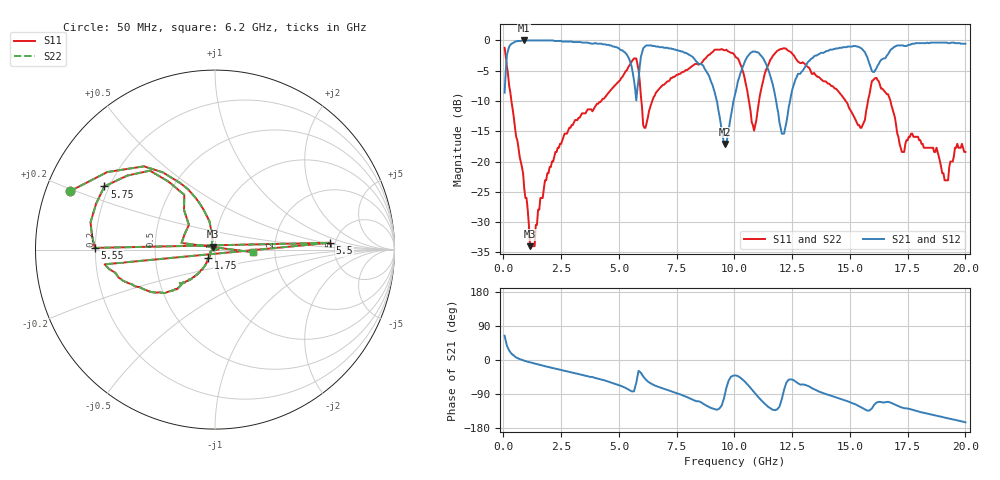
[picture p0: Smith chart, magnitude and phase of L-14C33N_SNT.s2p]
#	mhz	s	ma	r	50
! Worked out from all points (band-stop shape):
!   400 points, 50 MHz to 20 GHz, reference 50 ohm
!   highest |S21| = 0.00 dB at 900 MHz (marker M1); lowest = -17.1 dB at 9.6 GHz (marker M2)
!   |S21| within 3 dB of the highest: 138.4 MHz to 5.437 GHz (5.298 GHz wide, 190 % of centre); 16.44 GHz to end of sweep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
!   lowest |S11| = -34.0 dB at 1.15 GHz (marker M3), VSWR 1.04, Z = 48.7 + j1.52 ohm
!   |S11| at or under -10 dB: 344.4 MHz to 4.231 GHz (3.887 GHz wide, 170 % of centre); 14.82 GHz to 15.78 GHz (964.8 MHz wide, 6.31 % of centre); 16.76 GHz to end of sweep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
!   |S22| runs from -34.0 to -1.2 dB; largest |S21 - S12| = 0
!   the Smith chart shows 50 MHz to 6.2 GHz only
!   S11 on the Smith chart (normalised r, x): 50 MHz: 0.07, +0.19; 1.75 GHz: 0.93, -0.09; 5.5 GHz: 4.48, +0.58; 5.55 GHz: 0.20, +0.01; 5.75 GHz: 0.18, +0.26; 6.2 GHz: 1.53, -0.05
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50  0.87 158.0  0.37 64.0  0.37 64.0  0.87 158.0
900  0.06 103.7  1 -1.8  1 -1.8  0.06 103.7
1150  0.02 128.6  1 -6.3  1 -6.3  0.02 128.6
1750  0.06 -127.5  1 -15.7  1 -15.7  0.06 -127.5
3400  0.25 -132.7  0.96 -39.2  0.96 -39.2  0.25 -132.7
5450  0.62 -172.4  0.7 -79.3  0.7 -79.3  0.62 -172.4
5500  0.64 3.4  0.65 -81.0  0.65 -81.0  0.64 3.4
5550  0.67 179.2  0.61 -82.7  0.61 -82.7  0.67 179.2
5750  0.71 150.3  0.32 -60.3  0.32 -60.3  0.71 150.3
6200  0.21 -4.0  0.91 -53.7  0.91 -53.7  0.21 -4.0
6700  0.39 -172.2  0.89 -70.7  0.89 -70.7  0.39 -172.2
7050  0.45 -179.2  0.87 -78.3  0.87 -78.3  0.45 -179.2
7100  0.46 -0.1  0.87 -79.2  0.87 -79.2  0.46 -0.1
7150  0.46 179.0  0.86 -80.0  0.86 -80.0  0.46 179.0
7250  0.49 177.1  0.86 -82.4  0.86 -82.4  0.49 177.1
9600  0.83 104.6  0.14 -87.2  0.14 -87.2  0.83 104.6
10050  0.73 86.7  0.37 -40.7  0.37 -40.7  0.73 86.7
10850  0.18 104.9  0.81 -84.6  0.81 -84.6  0.18 104.9
12050  0.85 91.9  0.17 -103.3  0.17 -103.3  0.85 91.9
13350  0.53 42.8  0.71 -74.1  0.71 -74.1  0.53 42.8
16700  0.34 -6.7  0.8 -111.3  0.8 -111.3  0.34 -6.7
20000  0.12 -80.7  0.94 -164.5  0.94 -164.5  0.12 -80.7
